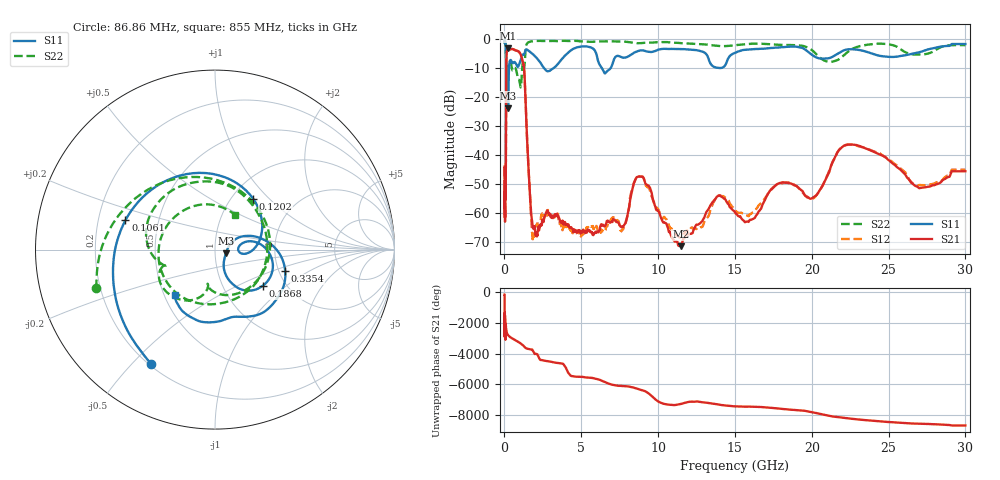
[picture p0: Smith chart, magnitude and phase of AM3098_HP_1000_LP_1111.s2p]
! Date/Time: Thu, Feb 28, 2019 8:40 AM
! Network Analyzer: Agilent Technologies E8364B Rev: A.07.50.67
! Sweep from 0.010 to 30.000 GHz, 1601 Points, Sweep Type: LOG
! Power Supply: 5.023 V, 0.002 A
# Hz S DB R 50
!freq MagS11 AngS11 MagS21 AngS21 MagS12 AngS12 MagS22 AngS22
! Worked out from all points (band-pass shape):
!   1601 points, 10 MHz to 30 GHz, reference 50 ohm
!   highest |S21| = -3.11 dB at 239.9 MHz (marker M1); lowest = -71.3 dB at 11.48 GHz (marker M2)
!   |S21| within 3 dB of the highest: 128 MHz to 1.112 GHz (983.5 MHz wide, 159 % of centre)
!   lowest |S11| = -23.8 dB at 238.7 MHz (marker M3), VSWR 1.14, Z = 56.5 - j2.22 ohm
!   |S11| at or under -10 dB: 192.4 MHz to 297.9 MHz (105.4 MHz wide, 43 % of centre); 2.602 GHz to 3.17 GHz (567.8 MHz wide, 19.7 % of centre); 6.355 GHz to 6.894 GHz (538.9 MHz wide, 8.14 % of centre)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
!   |S22| runs from -16.5 to -0.5 dB; largest |S21 - S12| = 0.011
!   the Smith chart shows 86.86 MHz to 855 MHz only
!   S11 on the Smith chart (normalised r, x): 86.86 MHz: 0.21, -0.57; 106.1 MHz: 0.32, +0.14; 120.2 MHz: 1.25, +0.81; 186.8 MHz: 1.53, -0.70; 335.4 MHz: 2.17, -0.61; 855 MHz: 0.57, -0.32
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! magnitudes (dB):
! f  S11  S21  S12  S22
! 10 MHz  -0.3  -43.9  -44.2  -0.6
! 38.04 MHz  -0.5  -62.1  -60.2  -1.0
! 86.86 MHz  -2.8  -53.2  -51.9  -3.2
! 106.1 MHz  -5.6  -25.8  -25.5  -7.3
! 120.2 MHz  -9.0  -9.5  -9.5  -10.7
! 144.7 MHz  -16.9  -4.3  -4.2  -13.3
! 186.8 MHz  -9.5  -3.6  -3.6  -8.9
! 238.7 MHz  -23.8  -3.1  -3.1  -10.9
! 239.9 MHz  -23.8  -3.1  -3.1  -10.9
! 335.4 MHz  -7.8  -3.4  -3.4  -7.8
! 550.5 MHz  -8.1  -3.4  -3.3  -10.7
! 855 MHz  -9.4  -4.0  -3.9  -13.0
! 1.27 GHz  -5.3  -9.7  -9.7  -9.9
! 1.784 GHz  -4.8  -62.0  -65.7  -0.6
! 2.084 GHz  -6.3  -67.4  -65.1  -0.5
! 7.926 GHz  -6.2  -62.3  -62.7  -0.8
! 8.893 GHz  -3.8  -47.3  -47.4  -1.3
! 11.48 GHz  -3.3  -71.3  -68.1  -1.3
! 13.88 GHz  -9.8  -54.1  -54.0  -2.2
! 20.1 GHz  -5.6  -54.5  -54.8  -4.1
! 22.56 GHz  -3.4  -36.2  -36.3  -3.5
! 30 GHz  -1.6  -45.5  -44.9  -2.0
